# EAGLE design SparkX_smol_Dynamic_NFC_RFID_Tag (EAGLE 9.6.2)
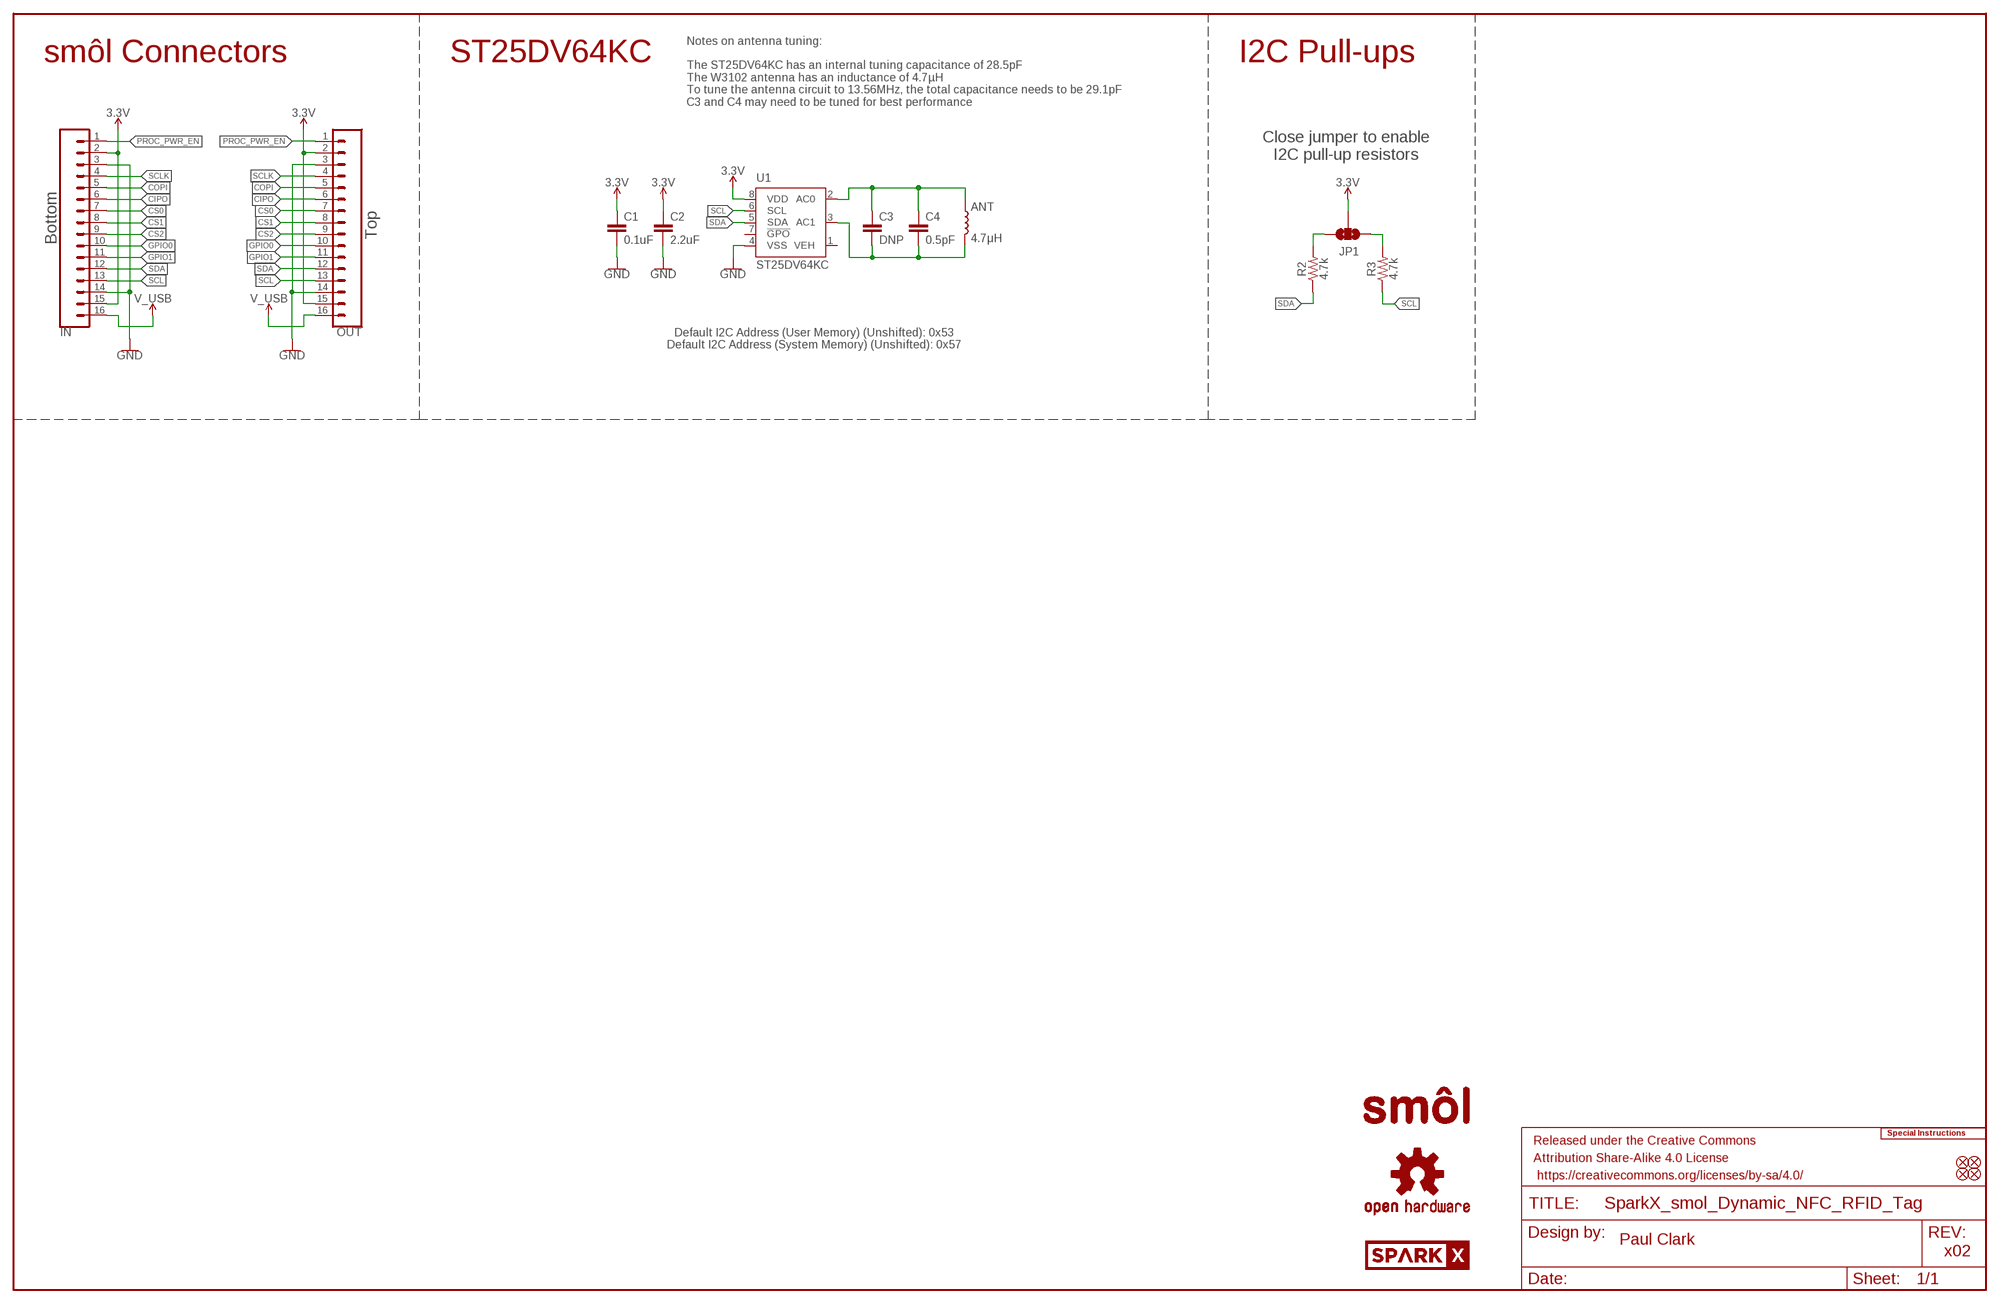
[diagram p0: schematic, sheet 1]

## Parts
ANT  4.7μH  RFID_ANTENNA_W3102  [W3102]
C1  0.1uF  0.1UF-0402T-6.3V-10%-X7R  [0402-TIGHT]
C2  2.2uF  2.2UF-0402_TIGHT-10V-10%-X5R  [0402-TIGHT]
C3  DNP  DNP-0402-TIGHT_NO_CREAM  [0402-TIGHT_NO_CREAM]
C4  0.5pF  0.5PF-0402_TIGHT-50V-PM0.05PF-NP0  [0402-TIGHT]
FD1  FIDUCIALUFIDUCIAL  [FIDUCIAL-MICRO]
FD2  FIDUCIALUFIDUCIAL  [FIDUCIAL-MICRO]
FD3  FIDUCIALUFIDUCIAL  [FIDUCIAL-MICRO]
FD4  FIDUCIALUFIDUCIAL  [FIDUCIAL-MICRO]
FRAME1  FRAME-LEDGER  [CREATIVE_COMMONS]
IN  CONN_16FPC_16_0.5MM  [FPC_16_0.5MM]
JP1  JUMPER-SMT_3_NO_SILK  [SMT-JUMPER_3_NO_SILK]
LOGO1  SPECIAL_INSTRUCTIONS-ORDERING  [ORDERING_INSTRUCTIONS]
LOGO2  OSHW-LOGOMINI  [OSHW-LOGO-MINI]
LOGO3  OSHW-LOGOMINI  [OSHW-LOGO-MINI]
OUT  CONN_16FPC_16_0.5MM  [FPC_16_0.5MM]
R2  4.7k  4.7KOHM-0402T-1/16W-1%  [0402-TIGHT]
R3  4.7k  4.7KOHM-0402T-1/16W-1%  [0402-TIGHT]
U1  ST25DV64KC  [SO08]
U$1  SPARKX-LOGO3  [SPARKX-SMALL]
U$3  SMOL_LOGOSMALL  [SMOL_SMALL]
U$9  SMOL_LOGOSMALL  [SMOL_SMALL]

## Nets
3.3V: C1.1 C2.1 IN.2 IN.15 JP1.2 OUT.2 OUT.15 U1.8(VDD)
CIPO: IN.6 OUT.6
COPI: IN.5 OUT.5
CS0: IN.7 OUT.7
CS1: IN.8 OUT.8
CS2: IN.9 OUT.9
GND: C1.2 C2.2 IN.3 IN.14 OUT.3 OUT.14 U1.4(VSS)
GPIO0: IN.10 OUT.10
GPIO1: IN.11 OUT.11
N$1: ANT.2 C3.2 C4.2 U1.3(AC1)
N$2: ANT.1 C3.1 C4.1 U1.2(AC0)
N$3: JP1.3 R2.2
N$4: JP1.1 R3.2
PROC_PWR_EN: IN.1 OUT.1
SCL: IN.13 OUT.13 R3.1 U1.6(SCL)
SCLK: IN.4 OUT.4
SDA: IN.12 OUT.12 R2.1 U1.5(SDA)
V_USB: IN.16 OUT.16
Unconnected: U1.7(!GPO!)

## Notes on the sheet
- Notes on antenna tuning:
  
  The ST25DV64KC has an internal tuning capacitance of 28.5pF
  The W3102 antenna has an inductance of 4.7µH
  To tune the antenna circuit to 13.56MHz, the total capacitance needs to be 29.1pF
  C3 and C4 may need to be tuned for best performance
- smôl Connectors | ST25DV64KC | I2C Pull-ups
- Close jumper to enable
  I2C pull-up resistors
- Top
- Bottom
- Default I2C Address (User Memory) (Unshifted): 0x53
  Default I2C Address (System Memory) (Unshifted): 0x57
- Paul Clark
- x02

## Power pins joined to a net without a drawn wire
VEH: U1.1(VEH)

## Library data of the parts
ANT = SparkFun-RF:RFID_ANTENNA_W3102: W3102 Pulse Larsen NFC / RFID SMD Antenna 13.56MHz 4.7μH; PROD_ID: ANT-16333
C1 = SparkFun-Capacitors:0.1UF: 0.1µF ceramic capacitors; PROD_ID: CAP-14993
C2 = SparkFun-Capacitors:2.2UF: 2.2µF ceramic capacitors; PROD_ID: CAP-14232
C3 = SparkFun-Capacitors:DNP: Do-Not-Populate capacitor
C4 = SparkFun-Capacitors:0.5PF: 0.5pF ceramic capacitors; PROD_ID: CAP-14362
FD1-FD4 = SparkFun-Aesthetics:FIDUCIAL: Fiducial Alignment Points
FRAME1 = SparkFun-Aesthetics:FRAME-LEDGER: Schematic Frame - Ledger
IN OUT = SparkFun-Connectors:CONN_16: Multi connection point. Often used as Generic Header-pin footprint for 0.1 inch spaced/style header connections On any of the 0.1 inch spaced packages, you can populate with these: Break Away Headers - Straight (PRT-00116) Break Away Male Headers - Right Angle (PRT-00553) Female Headers (PRT-00115)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; PROD_ID: CONN-16066
JP1 = SparkFun-Jumpers:JUMPER-SMT_3_NO: Normally open jumper This jumper has three pads in close proximity to each other. Apply solder to close the connection(s).
LOGO1 = SparkFun-Aesthetics:SPECIAL_INSTRUCTIONS: Special Ordering/Production Instructions Alert
LOGO2 LOGO3 = SparkFun-Aesthetics:OSHW-LOGO: Open-Source Hardware (OSHW) Logo
R2 R3 = SparkFun-Resistors:4.7KOHM: 4.7kΩ resistor; PROD_ID: RES-15343
U1 = SparkFun-RF:ST25DV64KC: Dynamic NFC/RFID Dynamic NFC/RFID tag IC with 4-Kbit, 16-Kbit or 64-Kbit EEPROM, fast transfer mode capability and optimized I2C.; PROD_ID: IC-16315
U$1 = SparkX:SPARKX-LOGO
U$3 U$9 = SparkX:SMOL_LOGO

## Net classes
1 Power: width 0.305 mm
2 3.3V: width 0.508 mm

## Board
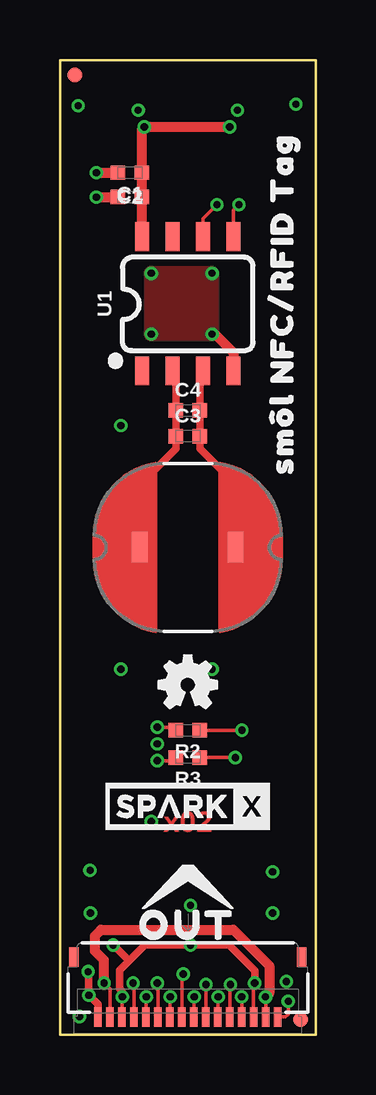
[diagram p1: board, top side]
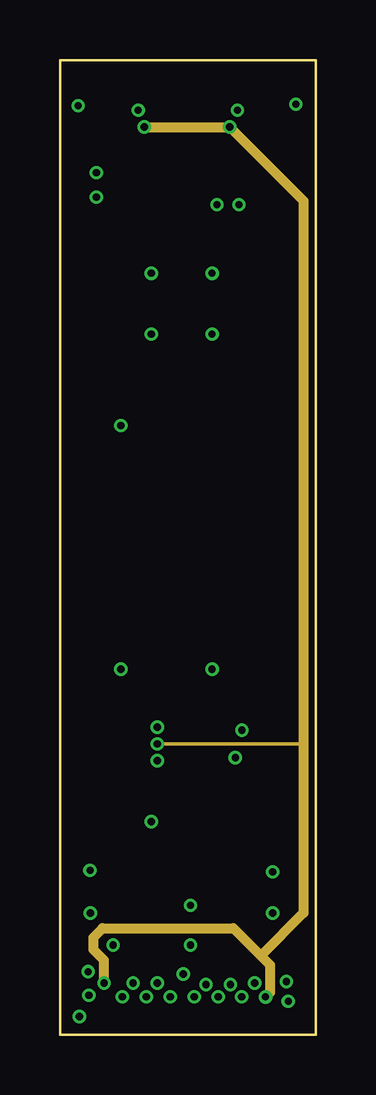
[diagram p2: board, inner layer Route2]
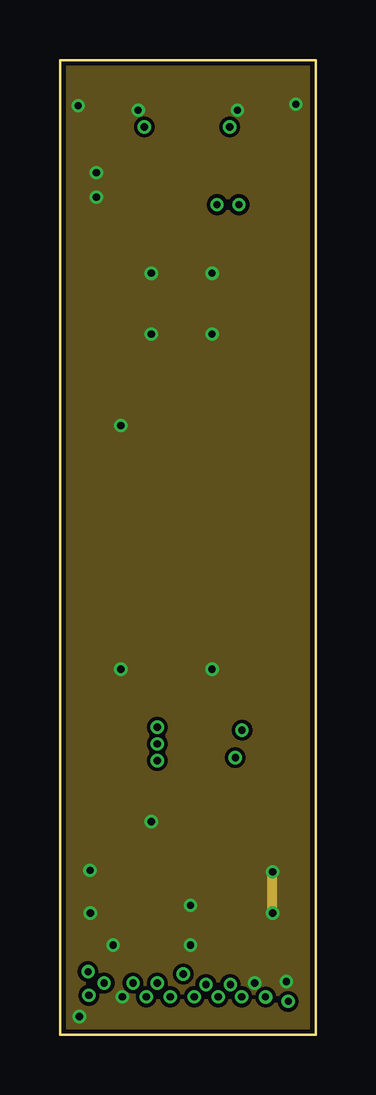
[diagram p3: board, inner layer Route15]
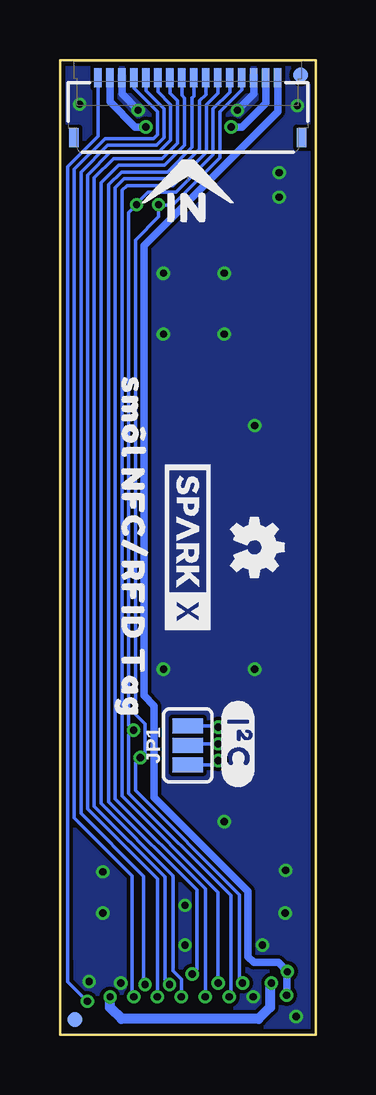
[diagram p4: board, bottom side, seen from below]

Size 10.67 x 40.64 mm. Coordinates in mm from the lower left corner, seen from the top.
Outline: 0,40.64 0,0 10.67,0 10.67,40.64 0,40.64
Copper layers (1+2*15+16): Top 0.035559375mm / dielectric 0.47751875mm / Route2 0.035559375mm / dielectric 0.47751875mm / Route15 0.035559375mm / dielectric 0.47751875mm / Bottom 0.035559375mm
Design rules "SparkFun-4-Layer-Minimum-JLCPCB *": minimum track width 5mil, minimum drill 0.2mm, track to track 5mil, track to pad 5mil, pad to pad 5mil, via to via 5mil, smd to smd 5mil, copper to edge 7mil, drill to drill 7mil, minimum pad ring 5mil, minimum via ring 5mil, stop-mask expansion 2.5mil, vias tented up to drill 25mil, thermal gap 10mil

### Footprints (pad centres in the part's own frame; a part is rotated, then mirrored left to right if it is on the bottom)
W3102 = smd 1.27 x 0.635: 1 0,2; 2 0,-2
0402-TIGHT = smd 0.6 x 0.6: 1 -0.5,0; 2 0.5,0
0402-TIGHT_NO_CREAM = smd 0.6 x 0.6: 1 -0.5,0; 2 0.5,0
FIDUCIAL-MICRO = smd 0.635 x 0.635: 1 0,0
FPC_16_0.5MM = smd 0.3 x 0.8: 1 -3.75,1.35; 2 -3.25,1.35; 3 -2.75,1.35; 4 -2.25,1.35; 5 -1.75,1.35; 6 -1.25,1.35; 7 -0.75,1.35; 8 -0.25,1.35; 9 0.25,1.35; 10 0.75,1.35; 11 1.25,1.35; 12 1.75,1.35; 13 2.25,1.35; 14 2.75,1.35; 15 3.25,1.35; 16 3.75,1.35 | smd 0.4 x 0.8: MP1 -4.75,-1.15; MP2 4.75,-1.15
SMT-JUMPER_3_NO_SILK = smd 0.635 x 1.27: 1 -0.813,0; 2 0,0; 3 0.813,0
SO08 = smd 0.6 x 1.2: 1 -1.905,-2.8; 2 -0.635,-2.8; 3 0.635,-2.8; 4 1.905,-2.8; 5 1.905,2.8; 6 0.635,2.8; 7 -0.635,2.8; 8 -1.905,2.8

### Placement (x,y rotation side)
ANT  5.33,20.32 90 top
C1  2.92,35.94 180 top
C2  2.92,34.92 180 top
C3  5.33,24.96 0 top
C4  5.33,26.04 0 top
FD1  0.64,40.01 0 top
FD2  0.64,40.01 0 bottom
FD3  10.03,0.64 0 top
FD4  10.03,0.64 0 bottom
FRAME1  not placed on the board
IN  5.33,38.54 0 bottom
JP1  5.33,12.06 90 bottom
LOGO1  not placed on the board
LOGO2  5.33,14.61 0 top
LOGO3  2.54,20.32 270 bottom
OUT  5.33,2.1 180 top
R2  5.33,12.7 180 top
R3  5.33,11.56 180 top
U1  5.33,30.48 0 top
U$1  5.33,9.53 0 top
U$2  [SM�L_NFC#RFID_TAG0]  9.27,30.48 90 top
U$3  5.33,6.41 0 top
U$4  [SM�L_NFC#RFID_TAG0]  7.62,20.32 270 bottom
U$5  [#I�C#0]  3.24,12.13 270 bottom
U$8  [IN0]  5.33,34.48 0 bottom
U$9  5.33,35.81 0 bottom
U$17  [OUT0]  5.33,4.57 0 top
U$20  SPARKX-LOGO3  [SPARKX-SMALL]  5.33,20.32 270 bottom

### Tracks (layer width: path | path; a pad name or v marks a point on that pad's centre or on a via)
3.3V  (via drill 0.3)
  Top 0.152: OUT.2 v8.58,1.58 | OUT.15 2.08,1.92 v1.84,2.16
  Top 0.406: v8.58,1.58 8.73,1.73 8.73,2.88 7.24,4.38 1.71,4.38 1.46,4.13 1.46,3.49 1.84,3.11 v1.84,2.16 | v7.08,37.85 v3.52,37.85 3.42,37.75 C1.1 C2.1 U1.8
  Route2 0.152: v4.06,12.13 10.16,12.13
  Route2 0.406: v1.84,2.16 1.84,3.11 1.4,3.56 1.4,4.06 1.78,4.45 7.24,4.45 8.38,3.3 | v8.58,1.58 8.76,1.77 8.76,2.92 8.38,3.3 | v3.52,37.85 v7.08,37.85 10.16,34.77 10.16,12.13 10.16,5.08 8.38,3.3
  Bottom 0.152: v4.06,12.13 5.27,12.13 JP1.2
  Bottom 0.305: IN.15 2.08,38.84 3.08,37.85 v3.52,37.85 | v7.08,37.85 7.53,37.85 8.58,38.9 IN.2
  Bottom 0.406: v1.84,2.16 1.91,2.1 1.91,1.14 2.38,0.66 8.1,0.66 8.58,1.14 v8.58,1.58
CIPO  (via drill 0.3)
  Top 0.152: OUT.6 6.58,1.57 v6.6,1.59
  Bottom 0.152: IN.6 6.58,39.32 6.05,38.78 6.05,37.29 6.53,36.81 8.55,36.81 9.51,35.85 9.51,9.41 6.6,6.5 v6.6,1.59
COPI  (via drill 0.3)
  Top 0.152: OUT.5 7.08,2.07 v7.11,2.1
  Bottom 0.152: IN.5 7.08,39.36 6.33,38.6 6.33,37.4 6.64,37.09 8.67,37.09 9.79,35.96 9.79,9.23 7.18,6.62 7.18,2.16 v7.11,2.1
CS0  (via drill 0.3)
  Top 0.152: OUT.7 6.08,2.08 v6.1,2.1
  Bottom 0.152: IN.7 6.08,39.26 5.77,38.94 5.77,37.17 6.41,36.53 8.44,36.53 9.23,35.73 9.23,9.53 6.29,6.58 6.29,2.29 v6.1,2.1
CS1  (via drill 0.3)
  Top 0.152: OUT.8 5.58,1.57 v5.6,1.59
  Bottom 0.152: IN.8 5.58,39.16 5.46,39.04 5.46,37.09 6.3,36.25 8.22,36.25 8.95,35.52 8.95,9.64 5.94,6.63 5.94,2.66 5.6,2.32 v5.6,1.59
CS2  (via drill 0.3)
  Top 0.152: OUT.9 5.08,2.48 v5.14,2.54
  Bottom 0.152: IN.9 5.08,39.13 5.15,39.07 5.15,37 6.18,35.97 8.11,35.97 8.64,35.44 8.64,9.72 4.95,6.04 4.95,2.73 v5.14,2.54
GND  (via drill 0.3)
  Top 0.152: v8.13,2.16 8.06,2.1 8.06,0.77 OUT.3 | OUT.14 2.58,1.57 v2.6,1.59
  Top 0.305: v2.6,1.59 2.6,1.82 2.49,1.93 2.49,2.68 2.89,3.08 | v8.13,2.16 8.13,2.67 7.05,3.75 3.56,3.75 2.89,3.08 | v2.22,3.75 2.89,3.08
  Top 0.406: v1.52,35.94 C1.2 | v1.52,34.92 C2.2 | v6.35,29.21 6.48,29.21 7.24,28.45 U1.4
  Route15 0.406: v8.88,5.08 v8.88,6.79
  Bottom 0.305: IN.14 2.58,39.23 v3.27,38.54 | IN.3 8.08,39.23 v7.4,38.54
  other vias: 1.27,5.08 9.84,38.8 0.76,38.73 9.45,2.22 6.35,31.75 3.81,29.21 3.81,31.75 2.54,15.24 6.35,15.24 3.81,8.89 2.54,25.4 1.25,6.86 0.81,0.76 5.45,3.75 5.45,5.4
  pour Bottom (isolate 0.152, rank 2): 0,40.64 10.67,40.64 10.67,0 0,0
  pour Route15 (isolate 0.152, rank 2): 0,40.64 10.67,40.64 10.67,0 0,0
  pour Top: 3.81,31.75 3.81,29.21 6.35,29.21 6.35,31.75
GPIO0  (via drill 0.3)
  Top 0.152: OUT.10 4.58,1.57 v4.6,1.59
  Bottom 0.152: IN.10 4.58,39.2 4.84,38.94 4.84,36.92 6.07,35.69 7.99,35.69 8.36,35.32 8.36,9.84 4.6,6.09 v4.6,1.59
GPIO1  (via drill 0.3)
  Top 0.152: OUT.11 4.08,2.14 v4.06,2.16
  Bottom 0.152: IN.11 4.08,39.26 4.56,38.78 4.56,36.8 5.95,35.41 7.87,35.41 8.08,35.21 8.08,9.95 4.06,5.94 v4.06,2.16
N$1
  Top 0.305: ANT.2 7.33,22.95 5.83,24.45 C3.2 C4.2 5.83,27.55 U1.3
N$2
  Top 0.305: U1.2 4.83,27.55 C4.1 C3.1 4.83,24.45 3.33,22.95 ANT.1
N$3  (via drill 0.3)
  Top 0.152: R2.2 4.71,12.83 v4.06,12.83
  Bottom 0.152: v4.06,12.83 4.12,12.88 JP1.3
N$4  (via drill 0.3)
  Top 0.152: R3.2 4.71,11.43 v4.06,11.43
  Bottom 0.152: v4.06,11.43 4.24,11.25 JP1.1
PROC_PWR_EN  (via drill 0.3)
  Top 0.152: v9.53,1.4 9.53,0.87 9.4,0.75 OUT.1
  Bottom 0.152: v9.53,1.4 10.35,2.22 10.35,3.11 10.35,36.2 9.08,37.46 IN.1
SCL  (via drill 0.3)
  Top 0.152: OUT.13 3.08,2.12 v3.05,2.16 | U1.6 5.97,34.02 v6.56,34.61 | v7.32,11.56 R3.1
  Bottom 0.152: IN.13 3.08,39.41 4,38.49 4,36.57 5.97,34.6 6.54,34.6 v6.56,34.61 6.56,34.1 7.52,33.14 7.52,13.36 7.11,12.95 7.11,11.76 v7.32,11.56 7.52,11.36 7.52,10.19 3.17,5.84 3.17,2.29 v3.05,2.16
SCLK  (via drill 0.3)
  Top 0.152: OUT.4 v7.58,1.59 | v7.58,1.59
  Bottom 0.152: IN.4 7.58,39.47 6.61,38.49 6.61,37.52 6.76,37.37 8.79,37.37 10.07,36.08 10.07,9.05 7.65,6.63 7.65,1.65 v7.58,1.59
SDA  (via drill 0.3)
  Top 0.152: OUT.12 3.58,1.57 v3.6,1.59 | U1.5 7.24,34.38 v7.47,34.61 | v7.6,12.7 R2.1
  Bottom 0.152: IN.12 3.58,39.3 4.28,38.6 4.28,36.69 5.83,35.13 7,35.13 7.47,34.66 v7.47,34.61 7.8,34.28 7.8,12.9 v7.6,12.7 7.8,12.5 7.8,10.07 3.54,5.81 3.54,1.65 v3.6,1.59
V_USB  (via drill 0.3)
  Top 0.305: OUT.16 1.58,1.27 v1.21,1.65 1.21,2.6 v1.18,2.63
  Bottom 0.305: v1.21,1.65 1.21,2.6 v1.18,2.63 1.56,3.02 2.57,3.02 2.82,3.26 2.82,5.99 6.73,9.9 6.73,13.71 7.16,14.14 7.16,32.9 1.58,38.48 IN.16

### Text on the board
Top: x02
Measures: Dimensions in Inches
tDocu: 4-Layer Board / 0.8mm Thickness / 1oz Copper (Outer layers) / HASL Finish | Paul Clark

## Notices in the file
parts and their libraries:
SparkFun-Aesthetics: Licensing: Creative Commons ShareAlike 4.0 International - https://creativecommons.org/licenses/by-sa/4.0
SparkFun-Aesthetics: Released under the Creative Commons Attribution Share-Alike 4.0 License
SparkFun-Aesthetics: https://creativecommons.org/licenses/by-sa/4.0
